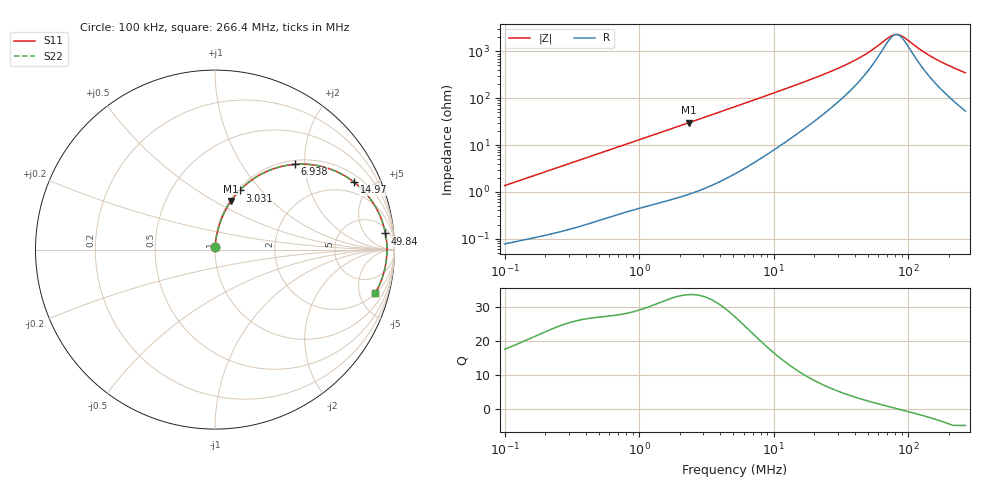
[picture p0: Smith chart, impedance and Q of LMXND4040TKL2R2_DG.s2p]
! LMXND4040TKL2R2_DG  S-PARAMETER MODEL  ( General Type )
! Model Generated by TAIYO YUDEN Corporation (http://www.ty-top.com)
! Version 1.0
! TAIYO YUDEN Control No. 191023NI43SB-FBB
! Copyright(c) 2019 TAIYO YUDEN CO.,LTD. All Rights Reserved.
! Product Description (link to TY-COMPAS)
! https://ds.yuden.co.jp/TYCOMPAS/or/detail?pn=LMXND4040TKL2R2MDG&u=M
! Products Name : Inductors
! Characteristics :
!  Inductance : 2.2 uH , SRF(min) : 60 MHz , DC Resistance(max) : 0.0504 Ohm
!  Rated Current : Saturation :3000 mA , Temp Rise : 2200 mA
!  Case Size : 4.0 x 4.0 / 0.157 x 0.157 [mm/inch] , Thickness : 1.8 / 0.071 [mm/inch]
!  (Conditions: Temperature = 25 degC , DC Bias Current/Voltage = 0A / 0V)
! External Node Assignments :
!  1  o---GGG---o  2
! GND o---------o GND
! Frequency Range : 0.1MHz  -  266.375554MHz  [ 402 STEP ]
# MHz S RI R 50
! Freq[MHz].  S11 Real  S11 Imag  S21 Real  S21 Imag  S12 Real  S12 Imag  S22 Real  S22 Imag
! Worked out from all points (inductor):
!   401 points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, 100 kHz to 266.4 MHz, reference 50 ohm
!   read as one part in series: L = 2.15 uH near 104 kHz
!   highest Q = 33.8 at 2.345 MHz (marker M1), where L = 2.03 uH
!   self-resonance near 81.81 MHz
!   S11 on the Smith chart (normalised r, x): 100 kHz: 1.00, +0.03; 3.031 MHz: 1.02, +0.77; 6.938 MHz: 1.08, +1.77; 14.97 MHz: 1.35, +3.91; 49.84 MHz: 8, +17; 266.4 MHz: 2.06, -6.89
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0.1  0.000955 0.0135  0.999 -0.0135  0.999 -0.0135  0.000955 0.0135
0.374775  0.00431 0.0492  0.9957 -0.0492  0.9957 -0.0492  0.00431 0.0492
0.762193  0.0132 0.0975  0.9868 -0.0975  0.9868 -0.0975  0.0132 0.0975
1.404561  0.0368 0.1729  0.9632 -0.1729  0.9632 -0.1729  0.0368 0.1729
2.345296  0.0892 0.2706  0.9108 -0.2706  0.9108 -0.2706  0.0892 0.2706
3.030584  0.1376 0.3297  0.8624 -0.3297  0.8624 -0.3297  0.1376 0.3297
3.994097  0.2138 0.3941  0.7862 -0.3941  0.7862 -0.3941  0.2138 0.3941
5.26394  0.3177 0.4473  0.6823 -0.4473  0.6823 -0.4473  0.3177 0.4473
6.937504  0.4436 0.4749  0.5564 -0.4749  0.5564 -0.4749  0.4436 0.4749
9.893512  0.6126 0.4581  0.3874 -0.4581  0.3874 -0.4581  0.6126 0.4581
14.96887  0.7743 0.3761  0.2257 -0.3761  0.2257 -0.3761  0.7743 0.3761
19.34272  0.8436 0.31  0.1564 -0.31  0.1564 -0.31  0.8436 0.31
32.94112  0.9241 0.1771  0.0759 -0.1771  0.0759 -0.1771  0.9241 0.1771
40.92036  0.9402 0.1298  0.0598 -0.1298  0.0598 -0.1298  0.9402 0.1298
49.83986  0.9496 0.0903  0.0504 -0.0903  0.0504 -0.0903  0.9496 0.0903
72.49162  0.9578 0.0214  0.0422 -0.0214  0.0422 -0.0214  0.9578 0.0214
80.00304  0.9583 0.00394  0.0417 -0.00394  0.0417 -0.00394  0.9583 0.00394
88.29277  0.9581 -0.0135  0.0419 0.0135  0.0419 0.0135  0.9581 -0.0135
125.9135  0.9519 -0.078  0.0481 0.078  0.0481 0.078  0.9519 -0.078
150.3647  0.9449 -0.1126  0.0551 0.1126  0.0551 0.1126  0.9449 -0.1126
202.1166  0.9248 -0.176  0.0752 0.176  0.0752 0.176  0.9248 -0.176
266.3756  0.8925 -0.2424  0.1075 0.2424  0.1075 0.2424  0.8925 -0.2424
